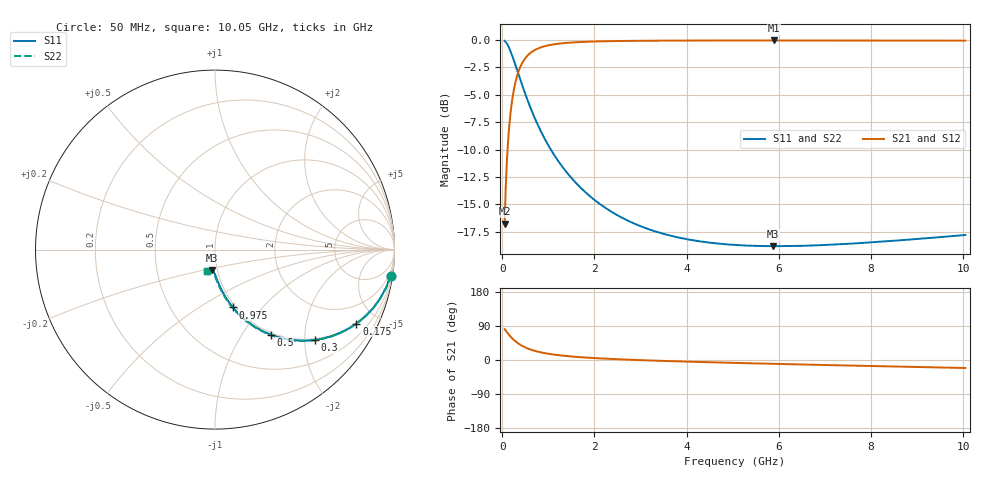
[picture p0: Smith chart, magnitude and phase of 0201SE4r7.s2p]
! AVX Thin Film Operation		Date: August 2001
! Description: Accu-P® Series, Thin Film, SMD, RF Capacitor
! Part Number: 0201ZK4R7ABW
! 50 MHz  -  10.05 GHz
! Serial Measurements
# mhz S db R 50
!	S11		S21		S12		S22
!	dB	Phase	dB	Phase	dB	Phase	dB	Phase
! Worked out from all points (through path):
!   401 points, 50 MHz to 10.05 GHz, reference 50 ohm
!   highest |S21| = -0.07 dB at 5.9 GHz (marker M1); lowest = -16.7 dB at 50 MHz (marker M2)
!   group delay of S21, straight-line fit = 13.8 ps
!   lowest |S11| = -18.8 dB at 5.875 GHz (marker M3), VSWR 1.26, Z = 47.1 - j10.8 ohm
!   |S11| at or under -10 dB: 1.053 GHz to end of sweep
!   |S22| runs from -18.8 to -0.1 dB; largest |S21 - S12| = 0
!   S11 on the Smith chart (normalised r, x): 50 MHz: 1, -13; 175 MHz: 0.97, -3.83; 300 MHz: 0.97, -2.24; 500 MHz: 0.97, -1.35; 975 MHz: 0.97, -0.71; 10.05 GHz: 0.89, -0.22
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50  -0.09 -8.5  -16.75 81.5  -16.75 81.5  -0.09 -8.5
75  -0.21 -12.6  -13.34 77.3  -13.34 77.3  -0.21 -12.7
125  -0.55 -20.5  -9.26 69.5  -9.26 69.5  -0.55 -20.6
175  -1.02 -27.6  -6.81 62.3  -6.81 62.3  -1.02 -27.7
225  -1.57 -34.0  -5.18 55.9  -5.18 55.9  -1.57 -34.1
300  -2.49 -42.1  -3.61 47.8  -3.61 47.8  -2.49 -42.3
400  -3.75 -50.5  -2.39 39.4  -2.39 39.4  -3.75 -50.7
500  -4.96 -56.8  -1.68 33.0  -1.68 33.0  -4.96 -57.1
600  -6.07 -61.7  -1.24 28.1  -1.24 28.1  -6.07 -62.1
700  -7.09 -65.5  -0.95 24.2  -0.95 24.2  -7.09 -65.9
975  -9.44 -72.7  -0.53 16.9  -0.53 16.9  -9.44 -73.3
1325  -11.69 -78.2  -0.31 11.3  -0.31 11.3  -11.69 -79.0
1725  -13.58 -82.2  -0.20 7.2  -0.20 7.2  -13.58 -83.2
2475  -15.93 -87.0  -0.12 2.2  -0.12 2.2  -15.93 -88.3
3400  -17.55 -91.0  -0.08 -2.1  -0.08 -2.1  -17.56 -92.6
4175  -18.29 -93.7  -0.07 -4.9  -0.07 -4.9  -18.29 -95.4
5050  -18.69 -96.4  -0.07 -7.7  -0.07 -7.7  -18.69 -98.2
5875  -18.80 -98.8  -0.07 -10.1  -0.07 -10.1  -18.80 -100.5
5900  -18.80 -98.9  -0.07 -10.2  -0.07 -10.2  -18.80 -100.6
6725  -18.74 -101.1  -0.07 -12.5  -0.07 -12.5  -18.74 -102.8
8400  -18.34 -105.5  -0.07 -16.9  -0.07 -16.9  -18.34 -107.1
10050  -17.78 -109.8  -0.09 -21.1  -0.09 -21.1  -17.78 -111.2
